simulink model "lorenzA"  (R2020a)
settings: Solver=ode45  StartTime=0.0  StopTime=50  MaxStep=1e-2  RelTol=1e-3  EnableMultiTasking=on
libraries: simulink x3

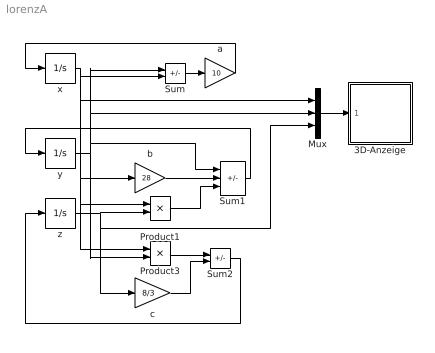
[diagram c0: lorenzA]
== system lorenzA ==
  note: .
  3D-Anzeige : Subsystem  mask(3D-Anzeige){phi=14, theta=14, psi=0, xlims=[-10,30], ylims=[-35,30], zlims=[0,50]}
      mask prompts: phi "Rollwinkel in Grad"; theta "Nickwinkel in Grad"; psi "Gierwinkel in Grad"; xlims "x-Bereich"; ylims "y-Bereich"; zlims "z-Bereich"
      mask help: Zeigt 3d-Vektor als Kurve im Raum, dargestellt in Dreitafelprojektion.
  Mux : Mux  Inputs=3
  Product1 : Product  InputSameDT=on  SaturateOnIntegerOverflow=on
  Product3 : Product  InputSameDT=on  SaturateOnIntegerOverflow=on
  Sum : Sum  Inputs=+-  InputSameDT=on  SaturateOnIntegerOverflow=on
  Sum1 : Sum  Inputs=-+-  InputSameDT=on  SaturateOnIntegerOverflow=on
  Sum2 : Sum  Inputs=+-  InputSameDT=on  SaturateOnIntegerOverflow=on
  a : Gain  Gain=10
  b : Gain  Gain=28
  c : Gain  Gain=8/3
  x : Integrator  InitialCondition=15
  y : Integrator  InitialCondition=15
  z : Integrator  InitialCondition=15
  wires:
  y/1 -> Product3/2, Sum/1, Mux/2, Sum1/1
  Sum/1 -> a/1
  x/1 -> Sum/2, Product1/1, Product3/1, b/1, Mux/1
  z/1 -> Product1/2, c/1, Mux/3
  b/1 -> Sum1/2
  Product1/1 -> Sum1/3
  Sum1/1 -> y/1
  a/1 -> x/1
  Product3/1 -> Sum2/1
  c/1 -> Sum2/2
  Sum2/1 -> z/1
  Mux/1 -> 3D-Anzeige/1(In)

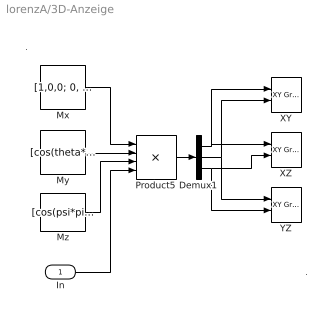
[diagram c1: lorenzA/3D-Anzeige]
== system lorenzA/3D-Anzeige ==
  note: .
  note: .
  In : Inport
  Demux1 : Demux  Outputs=3
  Mx : Constant  Value=[1,0,0; 0, cos(phi*pi/180), -sin(phi*pi/180); 0, sin(phi*pi/180), cos(phi*pi/180)]
  My : Constant  Value=[cos(theta*pi/180),0, sin(theta*pi/180); 0,1,0; -sin(theta*pi/180),0,cos(theta*pi/180)]
  Mz : Constant  Value=[cos(psi*pi/180),-sin(psi*pi/180), 0; sin(psi*pi/180), cos(psi*pi/180), 0; 0,0,1]
  Product5 : Product  Inputs=4  Multiplication=Matrix(*)  RndMeth=Zero
  XY : simulink/Sinks/XY Graph  xmin=xlims(1)  xmax=xlims(2)  ymin=ylims(1)  ymax=ylims(2)  st=-1
  XZ : simulink/Sinks/XY Graph  xmin=xlims(1)  xmax=xlims(2)  ymin=zlims(1)  ymax=zlims(2)  st=-1
  YZ : simulink/Sinks/XY Graph  xmin=ylims(1)  xmax=ylims(2)  ymin=zlims(1)  ymax=zlims(2)  st=-1
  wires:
  Demux1/1 -> XZ/1, XY/1
  In/1 -> Product5/4
  Mx/1 -> Product5/1
  My/1 -> Product5/2
  Mz/1 -> Product5/3
  Product5/1 -> Demux1/1
  Demux1/3 -> YZ/2, XZ/2
  Demux1/2 -> YZ/1, XY/2
